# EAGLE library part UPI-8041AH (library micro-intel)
MICROCOMPUTER/PERIPHERAL DEVICE
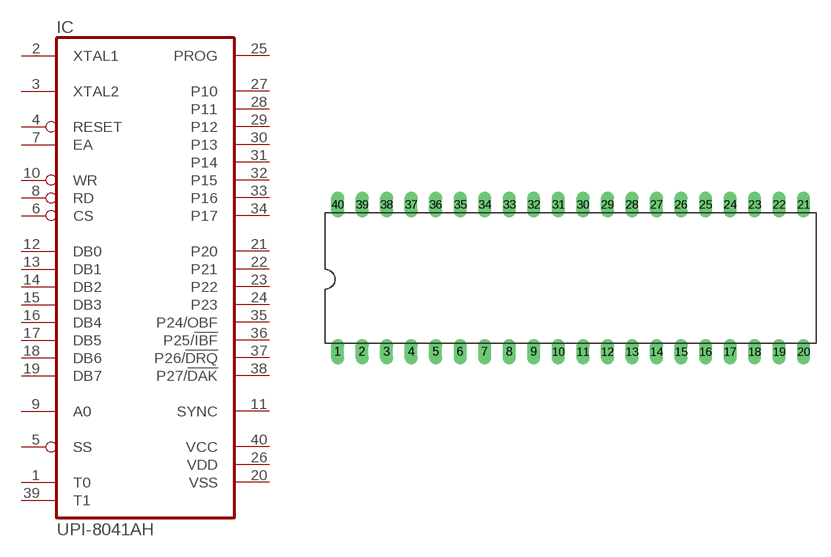
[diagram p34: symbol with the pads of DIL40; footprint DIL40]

Designator prefix IC

## UPI-8041AH (OC_FARNELL: unknown; OC_NEWARK: unknown)  [DIL40]
1  T0  in
2  XTAL1  in
3  XTAL2  in
4  RESET  in
5  SS  in
6  CS  in
7  EA  in
8  RD  in
9  A0  in
10  WR  in
11  SYNC  out
12  DB0
13  DB1
14  DB2
15  DB3
16  DB4
17  DB5
18  DB6
19  DB7
20  VSS  pwr
21  P20
22  P21
23  P22
24  P23
25  PROG
26  VDD  pwr
27  P10
28  P11
29  P12
30  P13
31  P14
32  P15
33  P16
34  P17
35  P24/OBF
36  P25/!IBF
37  P26/!DRQ
38  P27/!DAK
39  T1  in
40  VCC  pwr

## Footprint DIL40 (pad centres in mm)
Dual In Line Package
drill 0.813 long: 1 -24.13,-7.62; 2 -21.59,-7.62; 3 -19.05,-7.62; 4 -16.51,-7.62; 5 -13.97,-7.62; 6 -11.43,-7.62; 7 -8.89,-7.62; 8 -6.35,-7.62; 9 -3.81,-7.62; 10 -1.27,-7.62; 11 1.27,-7.62; 12 3.81,-7.62; 13 6.35,-7.62; 14 8.89,-7.62; 15 11.43,-7.62; 16 13.97,-7.62; 17 16.51,-7.62; 18 19.05,-7.62; 19 21.59,-7.62; 20 24.13,-7.62; 21 24.13,7.62; 22 21.59,7.62; 23 19.05,7.62; 24 16.51,7.62; 25 13.97,7.62; 26 11.43,7.62; 27 8.89,7.62; 28 6.35,7.62; 29 3.81,7.62; 30 1.27,7.62; 31 -1.27,7.62; 32 -3.81,7.62; 33 -6.35,7.62; 34 -8.89,7.62; 35 -11.43,7.62; 36 -13.97,7.62; 37 -16.51,7.62; 38 -19.05,7.62; 39 -21.59,7.62; 40 -24.13,7.62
